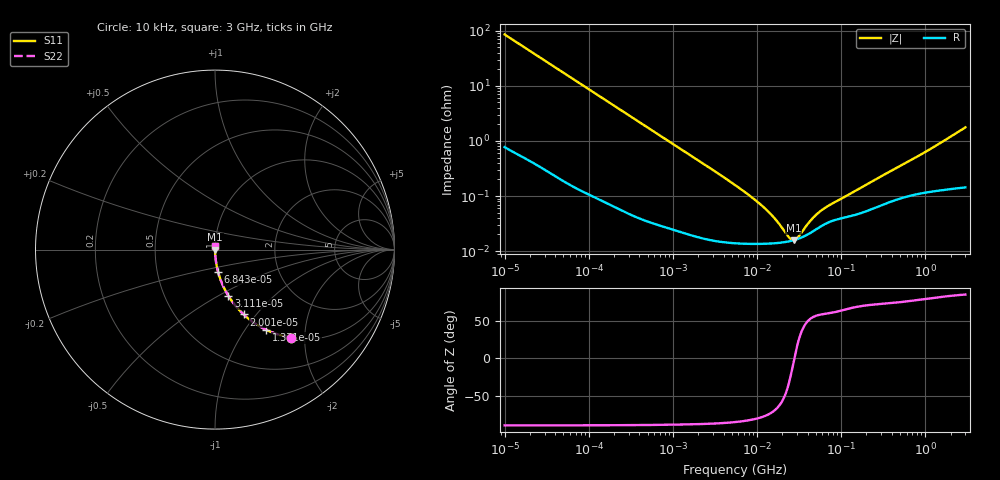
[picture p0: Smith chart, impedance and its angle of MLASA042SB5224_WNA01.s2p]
! MLASA042SB5224_WNA01  S-PARAMETER MODEL  ( Standard Model )
! Model Generated by TAIYO YUDEN Corporation (http://www.ty-top.com)
! Version 1.0
! TAIYO YUDEN Control No. 241206
! Copyright(c) 2024 TAIYO YUDEN CO.,LTD. All Rights Reserved.
! Product Description (link to TY-COMPAS)
! https://ds.yuden.co.jp/TYCOMPAS/or/detail?pn=MLASA042SB5224KWNA01&u=M
! Products Name : Multilayer Ceramic Capacitors
! Characteristics :
!  Capacitance : 0.22 [uF] , Rated Voltage : 4 [V] , TCC : X5R
!  Case Size : 0.4 x 0.2 / 0.016 x 0.008 [mm/inch] , Thickness : 0.2 / 0.008 [mm/inch]
!  (Conditions: Temperature = 25 [degC] , DC Bias Voltage = 0 [V])
! External Node Assignments :
!  1  o---| |---o  2
! GND o---------o GND
! Frequency Range : 10kHz  -  3GHz  [ 401 STEP ]
# MHZ S RI R 50
! Freq[MHz].  S11 Real  S11 Imag  S21 Real  S21 Imag  S12 Real  S12 Imag  S22 Real  S22 Imag
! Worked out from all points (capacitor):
!   401 points, 10 kHz to 3 GHz, reference 50 ohm
!   read as one part in series: C = 185 nF near 10.65 kHz
!   lowest |Z| = 15.8 mohm at 27.35 MHz (marker M1)
!   series resonance near 27.81 MHz, so ESL is about 180 pH
!   S11 on the Smith chart (normalised r, x): 10 kHz: 1.02, -1.72; 13.71 kHz: 1.01, -1.26; 20.01 kHz: 1.01, -0.86; 31.11 kHz: 1.01, -0.56; 68.43 kHz: 1.00, -0.25; 3 GHz: 1.00, +0.04
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0.01  0.4261 -0.49  0.5739 0.49  0.5739 0.49  0.4261 -0.49
0.013707  0.2852 -0.4468  0.7148 0.4468  0.7148 0.4468  0.2852 -0.4468
0.02001  0.1596 -0.3613  0.8404 0.3613  0.8404 0.3613  0.1596 -0.3613
0.031113  0.0743 -0.257  0.9257 0.257  0.9257 0.257  0.0743 -0.257
0.068432  0.0173 -0.1248  0.9827 0.1248  0.9827 0.1248  0.0173 -0.1248
0.082683  0.0122 -0.104  0.9878 0.104  0.9878 0.104  0.0122 -0.104
0.199902  0.00255 -0.0437  0.9974 0.0437  0.9974 0.0437  0.00255 -0.0437
0.683653  0.000461 -0.0129  0.9995 0.0129  0.9995 0.0129  0.000461 -0.0129
5.477226  0.000141 -0.00158  0.9999 0.00158  0.9999 0.00158  0.000141 -0.00158
8.789267  0.000136 -0.000923  0.9999 0.000923  0.9999 0.000923  0.000136 -0.000923
12.43293  0.000136 -0.00058  0.9999 0.00058  0.9999 0.00058  0.000136 -0.00058
16.51234  0.000139 -0.000354  0.9999 0.000354  0.9999 0.000354  0.000139 -0.000354
24.10585  0.00015 -9.3e-05  0.9998 9.3e-05  0.9998 9.3e-05  0.00015 -9.3e-05
25.67485  0.000154 -5.17e-05  0.9998 5.17e-05  0.9998 5.17e-05  0.000154 -5.17e-05
27.34599  0.000157 -1.08e-05  0.9998 1.08e-05  0.9998 1.08e-05  0.000157 -1.08e-05
31.02164  0.000167 7.08e-05  0.9998 -7.08e-05  0.9998 -7.08e-05  0.000167 7.08e-05
45.28751  0.000223 0.000315  0.9998 -0.000315  0.9998 -0.000315  0.000223 0.000315
54.71863  0.000268 0.000431  0.9997 -0.000431  0.9997 -0.000431  0.000268 0.000431
68.23149  0.000324 0.000558  0.9997 -0.000558  0.9997 -0.000558  0.000324 0.000558
374.4521  0.000777 0.00264  0.9992 -0.00264  0.9992 -0.00264  0.000777 0.00264
964.2293  0.00117 0.00598  0.9988 -0.00598  0.9988 -0.00598  0.00117 0.00598
3000  0.00174 0.0175  0.9983 -0.0175  0.9983 -0.0175  0.00174 0.0175
